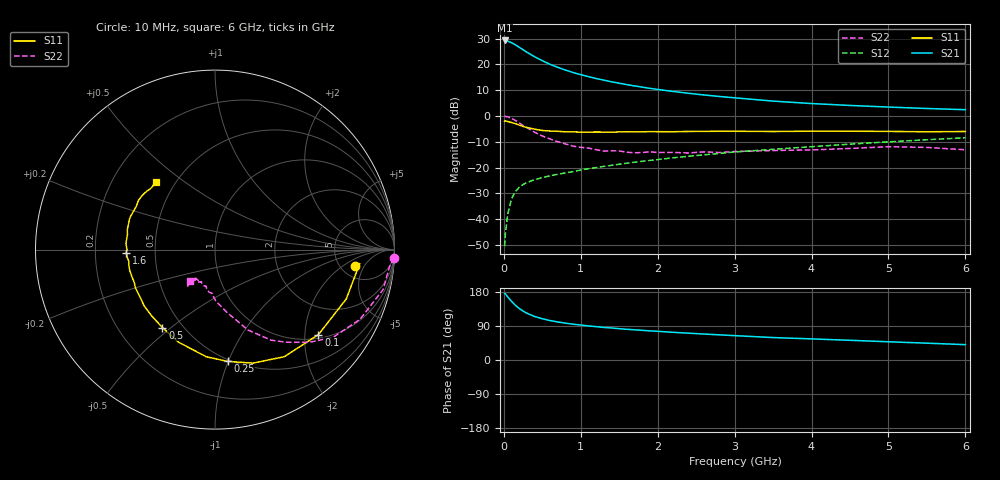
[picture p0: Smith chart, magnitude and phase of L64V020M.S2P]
!  INFINEON TECHNOLOGIES Small Signal Semiconductors
! BFR380L3 , Si-NPN RF-Transistor in TSLP-3-1
!  Vce=4 V,  Ic=20 mA
! Common Emitter S-Parameters:  07. March 2005
#  GHz  S  MA  R  50
! f  S11  S21  S12  S22
! GHz  Mag  Ang  Mag  Ang  Mag  Ang  Mag  Ang
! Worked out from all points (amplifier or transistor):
!   36 points, 10 MHz to 6 GHz, reference 50 ohm
!   highest |S21| = 29.3 dB at 10 MHz (marker M1)
!   |S21| within 3 dB of that: start of sweep to 219.1 MHz
!   unconditionally stable (mu >= 1): 2.13 GHz to 4.744 GHz
!   at 250 MHz: K = 0.33, MSG = 26.1 dB, |S12| = -26.6 dB
!   at 1.4 GHz: K = 0.92, MSG = 16.2 dB, |S12| = -19.1 dB
!   at 6 GHz: K = 0.97, MSG = 5.4 dB, |S12| = -8.4 dB
!   S11 on the Smith chart (normalised r, x): 10 MHz: 6.76, -3.16; 100 MHz: 1.10, -2.35; 250 MHz: 0.48, -0.99; 500 MHz: 0.39, -0.47; 1.6 GHz: 0.34, -0.01; 6 GHz: 0.39, +0.40
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0.01  0.7841 -6.6  29.05 175.3  0.003 81.6  0.9997 -2.7
0.02  0.8103 -5.5  28.74 174.7  0.0052 91.4  0.9772 -5.5
0.05  0.7812 -20.6  28.21 166.7  0.0126 82.1  0.9625 -13.4
0.1  0.746 -39.4  26.27 154.8  0.0249 71.7  0.8963 -25.7
0.15  0.7108 -57.1  23.96 144.3  0.0342 64.2  0.8192 -36.7
0.2  0.667 -71.5  21.45 135.9  0.0414 60.5  0.7358 -44.6
0.25  0.6266 -83.6  19.21 129.2  0.0469 56.0  0.6535 -52.2
0.3  0.5989 -94.7  17.16 123.4  0.0516 53.9  0.594 -58.2
0.4  0.5542 -111.6  14.05 114.8  0.0581 51.6  0.4833 -67.8
0.5  0.5238 -124.0  11.76 108.9  0.0642 51.1  0.4098 -73.3
0.6  0.5106 -134.1  10.02 104.1  0.069 51.0  0.3586 -79.0
0.7  0.5041 -141.4  8.761 100.4  0.0743 52.3  0.3182 -83.9
0.9  0.492 -154.3  6.946 94.5  0.0834 54.1  0.2602 -92.2
1.1  0.487 -162.3  5.773 89.9  0.095 55.8  0.2392 -98.0
1.4  0.4841 -172.0  4.595 84.5  0.1104 57.9  0.2114 -104.8
1.6  0.4946 -178.1  4.045 81.0  0.1217 59.0  0.1982 -112.6
2.2  0.4947 170.4  2.989 73.1  0.1546 61.1  0.1967 -117.6
2.8  0.5059 160.4  2.389 66.4  0.1877 62.3  0.1961 -125.3
3.5  0.5003 151.2  1.941 59.2  0.226 61.3  0.2143 -125.9
4.5  0.5064 144.5  1.598 52.0  0.2845 60.7  0.2346 -126.8
5.5  0.494 136.1  1.396 44.4  0.3462 57.9  0.2457 -127.2
6  0.5001 130.9  1.323 40.5  0.3787 56.1  0.2212 -128.4
